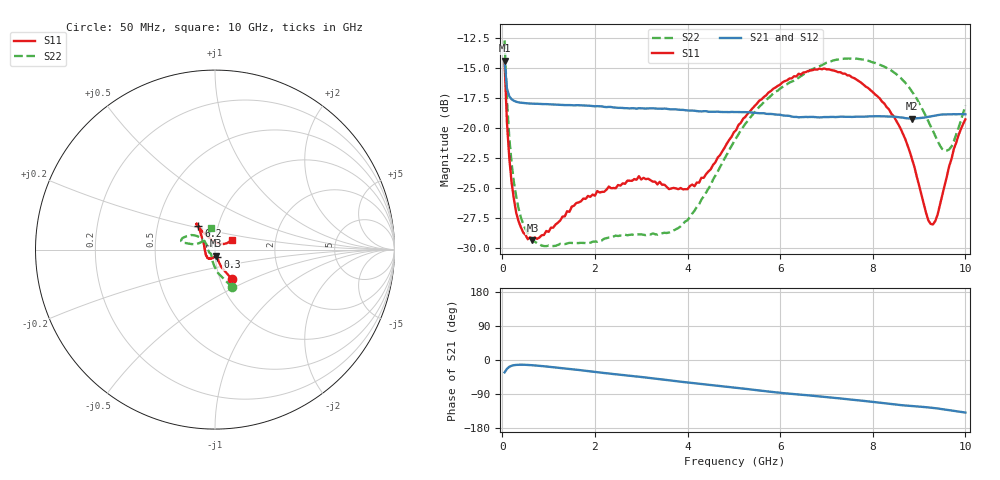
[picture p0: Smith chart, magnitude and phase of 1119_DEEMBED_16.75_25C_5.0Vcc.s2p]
!Hittite Microwave Corp.
!Digital Attenuator/PhaseShifter Rev 1.4.0
!Filename: C:\DATA\DATA\1119_DEEMBED_16.75_25C_5.0Vcc.s2p
!VNA ID: Agilent Technologies,N5224A,MY51441122,A.10.45.03
!Device type:
!2 Port Calibration.
!Temp(C): 25
!Lot Number:
!Serial Number:
!Operator:
!Misc:
!Attenuator:  16.750
# GHZ S DB R 50.0
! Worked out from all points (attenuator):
!   200 points, 50 MHz to 10 GHz, reference 50 ohm
!   highest |S21| = -14.38 dB at 50 MHz (marker M1); lowest = -19.2 dB at 8.85 GHz (marker M2)
!   lowest |S11| = -29.4 dB at 650 MHz (marker M3), VSWR 1.07, Z = 50.6 - j3.37 ohm
!   |S11| at or under -10 dB: start of sweep to end of sweep
!   |S22| runs from -29.9 to -12.7 dB; largest |S21 - S12| = 0.00034
!   S11 on the Smith chart (normalised r, x): 50 MHz: 1.14, -0.38; 300 MHz: 1.02, -0.09; 6.2 GHz: 0.80, +0.22; 10 GHz: 1.20, +0.14
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0.05  -14.55 -60.4  -14.38 -32.5  -14.38 -32.5  -12.68 -65.3
0.1  -19.50 -69.7  -16.69 -23.4  -16.68 -23.4  -17.62 -82.7
0.15  -22.45 -72.4  -17.34 -18.1  -17.34 -18.1  -20.75 -92.4
0.3  -27.07 -72.9  -17.80 -12.9  -17.80 -12.9  -25.71 -109.3
0.45  -28.72 -72.9  -17.90 -12.5  -17.90 -12.5  -28.00 -119.8
0.65  -29.37 -78.1  -17.96 -13.8  -17.96 -13.8  -29.32 -128.3
1.75  -25.89 -109.6  -18.11 -27.8  -18.11 -27.8  -29.60 -138.2
2.95  -24.02 -131.1  -18.34 -44.1  -18.35 -44.2  -28.89 -157.2
3.4  -24.49 -148.6  -18.38 -50.6  -18.38 -50.6  -28.84 -170.4
4.15  -24.86 173.5  -18.55 -61.4  -18.56 -61.4  -26.91 158.9
5.05  -20.17 137.2  -18.66 -73.1  -18.68 -73.2  -20.84 140.4
5.55  -17.71 129.3  -18.76 -80.3  -18.77 -80.4  -18.22 142.7
6.2  -15.86 125.0  -18.98 -89.2  -19.00 -89.2  -16.20 148.4
6.7  -15.16 125.5  -19.07 -94.4  -19.08 -94.4  -15.07 155.0
7.5  -15.61 126.8  -19.06 -104.1  -19.07 -104.2  -14.19 164.0
8.35  -18.44 124.1  -19.04 -115.4  -19.04 -115.4  -15.08 167.6
8.85  -22.63 115.7  -19.21 -121.5  -19.21 -121.5  -16.97 167.0
9.2  -27.72 83.8  -19.06 -125.1  -19.08 -125.2  -19.45 162.9
9.3  -28.05 65.0  -18.99 -126.4  -19.01 -126.5  -20.24 158.8
9.5  -25.61 37.9  -18.87 -129.7  -18.88 -129.7  -21.75 143.3
9.65  -23.18 29.4  -18.85 -132.3  -18.86 -132.3  -21.78 126.7
10  -19.27 31.1  -18.85 -138.7  -18.86 -138.7  -18.12 99.5
